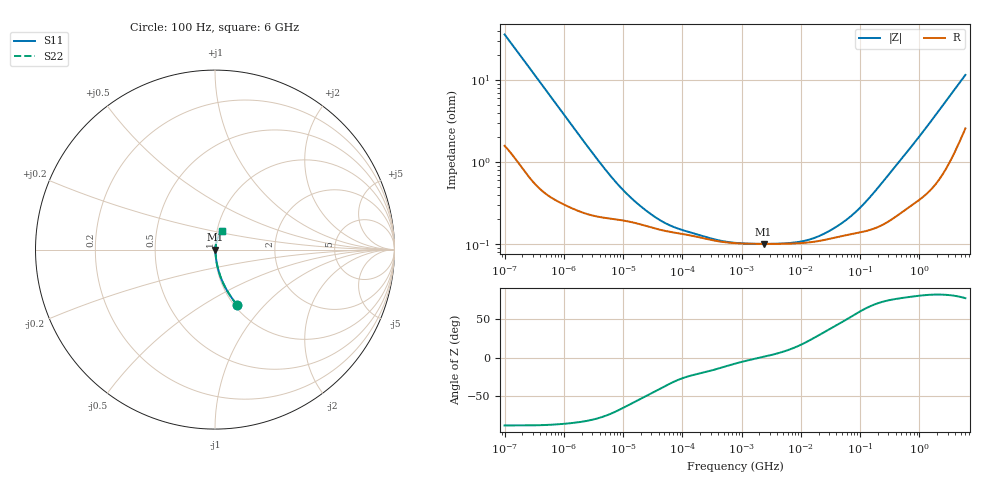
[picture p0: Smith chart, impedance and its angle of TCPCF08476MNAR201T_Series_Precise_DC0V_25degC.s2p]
! TCPCF08476MNAR201T Polymer Tantalum Capacitor Sparameter Model
! Model Generated by Samsung Electro-Mechanics
! Samsung Sparameter Version 5.0
! Date : Oct-21-2025
! Products : Polymer Tantalum Capacitor
! Characteristics :
!  Nominal Capacitance = 47uF
!  Capacitance Tolerance = +/-20%
!  ESR = 200 mohm max at 100kHz
!  Rated Voltage = 8Vdc
!  Size = 0805(unit:inch), 2012(unit:mm)
!  Length = 2.00+/-0.20mm
!  Width = 1.25+/-0.20mm
!  Thickness = 0.80+/-0.10mm
!  Lineup = Conductive Polymer Type
!  Feature = PCF
!  Measurement Temperature : 25degC.
!  DC bias Value = 0V
!  Frequency : 100Hz ~ 6GHz
! External Node Assignments :
!  1  o---||---o  2
# MHz S RI R 50.0
! Freq.  Real(S11)  Im(S11)  Real(S12)  Im(S12)  Real(S21)  Im(S21)  Real(S22)  Im(S22)
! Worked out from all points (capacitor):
!   300 points, 100 Hz to 6 GHz, reference 50 ohm
!   read as one part in series: C = 44.1 uF near 106.2 Hz
!   lowest |Z| = 101 mohm at 2.346 MHz (marker M1)
!   series resonance near 1.986 MHz, so ESL is about 150 pH
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0.0001  0.124 -0.3083  0.876 0.3083  0.876 0.3083  0.124 -0.3083
0.0001714451  0.0516 -0.1995  0.9484 0.1995  0.9484 0.1995  0.0516 -0.1995
0.0003517965  0.0158 -0.1029  0.9842 0.1029  0.9842 0.1029  0.0158 -0.1029
0.0007664292  0.0057 -0.0484  0.9943 0.0484  0.9943 0.0484  0.0057 -0.0484
0.001998454  0.00281 -0.0191  0.9972 0.0191  0.9972 0.0191  0.00281 -0.0191
0.004907976  0.00215 -0.00796  0.9979 0.00796  0.9979 0.00796  0.00215 -0.00796
0.009485389  0.00197 -0.00431  0.998 0.00431  0.998 0.00431  0.00197 -0.00431
0.01833192  0.00177 -0.00246  0.9982 0.00246  0.9982 0.00246  0.00177 -0.00246
0.03993819  0.00151 -0.00131  0.9985 0.00131  0.9985 0.00131  0.00151 -0.00131
0.06449105  0.0014 -0.000899  0.9986 0.000899  0.9986 0.000899  0.0014 -0.000899
0.1105667  0.00131 -0.00062  0.9987 0.00062  0.9987 0.00062  0.00131 -0.00062
0.366355  0.0011 -0.000291  0.9989 0.000291  0.9989 0.000291  0.0011 -0.000291
0.7981464  0.00103 -0.000131  0.999 0.000131  0.999 0.000131  0.00103 -0.000131
2.346024  0.00101 2.18e-05  0.999 -2.18e-05  0.999 -2.18e-05  0.00101 2.18e-05
7.321436  0.00102 0.000221  0.999 -0.000221  0.999 -0.000221  0.00102 0.000221
15.95059  0.00106 0.000491  0.9989 -0.000491  0.9989 -0.000491  0.00106 0.000491
34.75019  0.00118 0.00097  0.9988 -0.00097  0.9988 -0.00097  0.00118 0.00097
71.30563  0.00132 0.00177  0.9987 -0.00177  0.9987 -0.00177  0.00132 0.00177
129.7964  0.00146 0.00304  0.9985 -0.00304  0.9985 -0.00304  0.00146 0.00304
318.7652  0.00198 0.00703  0.998 -0.00703  0.998 -0.00703  0.00198 0.00703
1810.813  0.00639 0.0351  0.9936 -0.0351  0.9936 -0.0351  0.00639 0.0351
6000  0.0365 0.1054  0.9635 -0.1054  0.9635 -0.1054  0.0365 0.1054
